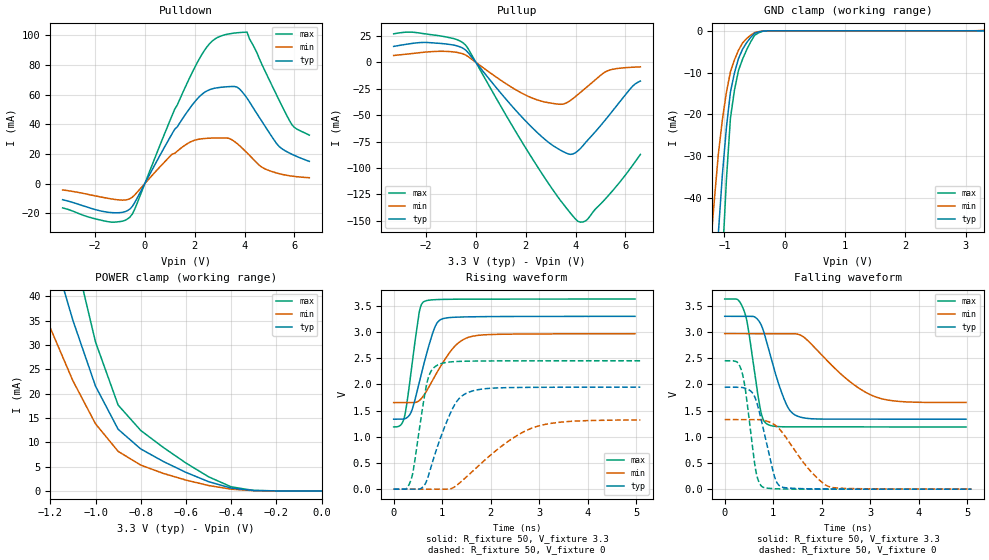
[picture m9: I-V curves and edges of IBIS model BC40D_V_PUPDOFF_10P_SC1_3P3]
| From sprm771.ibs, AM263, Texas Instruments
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|   Model Cell BC40D_V_PUPDOFF_10P_SC1_3P3
|BC40D_V_PUPDOFF_10P_SC1_3P3
[Model]   BC40D_V_PUPDOFF_10P_SC1_3P3
Model_type   I/O
Polarity   Non-Inverting
Enable   Active-Low
Vinl =  0.8V
Vinh =  2V
Cref =  15pF
Rref =  100.0000M
Vref =  0V
Vmeas =  1.65
C_comp   2.059994p   1.912853p   2.135747p
|[Input load] weak_pupdoff
|[Output drive] slow
|[supplytol] 10
|[temp] ind
[Model Spec]
Vinl   0.8V   0.8V   0.8V
Vinh   2V   2V   2V
[Temperature Range]   25   125   -40
[Voltage Range]   3.3   2.97   3.63
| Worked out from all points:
|   slope of the pulldown table from 0 to 0.495 V, typ, clamps not added: 31.8 ohm
|   slope of the pullup table from 0 to 0.495 V, typ, clamps not added: 33.8 ohm
|   GND clamp passes 1 mA (typ) near -0.53 V on its own axis
|   POWER clamp passes 1 mA (typ) near -0.43 V on its own axis
|   rising waveform, R_fixture 50, V_fixture 3.3: 20-80 % time 334ps typ, 531ps min, 209ps max; typ from 1.34 V to 3.3 V
|   rising waveform, R_fixture 50, V_fixture 0: 20-80 % time 466ps typ, 1.07ns min, 244ps max; typ from 0 V to 1.95 V
|   falling waveform, R_fixture 50, V_fixture 3.3: 20-80 % time 385ps typ, 931ps min, 234ps max; typ from 3.3 V to 1.34 V
|   falling waveform, R_fixture 50, V_fixture 0: 20-80 % time 293ps typ, 644ps min, 201ps max; typ from 1.95 V to 0 V
| Nom Voltages:
|   VDD=1.1001, VDDS=3.3, VDDS18=1.8, ESD_BIASFET=0, VSS=0, VSSS=0
| Min Voltages:
|   VDD=0.99, VDDS=2.97, VDDS18=1.62, ESD_BIASFET=0, VSS=0, VSSS=0
| Max Voltages:
|   VDD=1.21, VDDS=3.63, VDDS18=1.98, ESD_BIASFET=0, VSS=0, VSSS=0
[POWER_clamp]
|   voltage   I(typ)   I(min)   I(max)
-3.3V     446.9mA    419.5mA    603.9mA
-1.267V   62.17mA    41.5mA     88.03mA
-1.233V   56.52mA    37.5mA     80.22mA
-1.133V   40.34mA    26.27mA    57.61mA
-1.067V   30.56mA    19.7mA     43.68mA
-1.033V   26.05mA    16.75mA    37.15mA
-1V       21.55mA    13.8mA     30.62mA
-900mV    12.68mA    8.135mA    17.65mA
-800mV    8.63mA     5.309mA    12.43mA
-600mV    3.813mA    2.231mA    5.733mA
-400mV    580.7uA    357.1uA    842.6uA
0V        4.589uA    2.01uA     9.301uA
[Pulldown]
|   voltage   I(typ)   I(min)   I(max)
-3.3V     -10.93mA   -4.311mA   -16.48mA
-1.4V     -19.53mA   -10.23mA   -25.96mA
-600mV    -17.23mA   -10.26mA   -22.66mA
1.1V      33.82mA    19.89mA    46.25mA
2V        55.14mA    29.24mA    78.29mA
2.6V      63.35mA    30.61mA    94.45mA
3.2V      65.21mA    30.81mA    100.4mA
3.7V      65.09mA    27.02mA    101.8mA
4.1V      57.63mA    20.71mA    102.2mA
5.3V      26.68mA    7.058mA    59.31mA
5.9V      19.77mA    5.007mA    39.76mA
6.6V      14.97mA    3.923mA    32.7mA
[Pullup]
|   voltage   I(typ)   I(min)   I(max)
-3.3V     15.12mA    6.498mA    27.02mA
-1.9V     18.73mA    9.943mA    26.53mA
-900mV    16.4mA     9.888mA    22.58mA
-400mV    11.39mA    6.786mA    15.98mA
2.4V      -65.08mA   -35.06mA   -96.18mA
3.5V      -84.52mA   -39.53mA   -134mA
3.8V      -87.17mA   -36.01mA   -143mA
4.1V      -83.69mA   -30.35mA   -150.6mA
4.4V      -75.99mA   -24.42mA   -150.3mA
5.3V      -51.41mA   -7.872mA   -126.6mA
6.3V      -22.29mA   -4.606mA   -97.15mA
6.6V      -17.71mA   -4.277mA   -87.2mA
[GND_clamp]
|   voltage   I(typ)   I(min)   I(max)
-3.3V     -787.2mA   -607.8mA   -1.235A
-1.233V   -85.66mA   -52.14mA   -138.8mA
-1.167V   -66.47mA   -40.37mA   -107.7mA
-1.1V     -48.25mA   -29.37mA   -77.98mA
-1.033V   -34.27mA   -21.19mA   -54.56mA
-966.7mV  -23.06mA   -14.66mA   -35.51mA
-900mV    -14.61mA   -9.789mA   -20.83mA
-833.3mV  -10.05mA   -6.934mA   -14.15mA
-700mV    -4.416mA   -2.931mA   -6.811mA
-500mV    -621.6uA   -443.4uA   -1.094mA
-300mV    -17.13uA   -24.29uA   -23.57uA
3.3V      4.589uA    110.6uA    5.608uA
[Ramp]
| variable   typ   min   max
dV/dt_f  1.1805738/0.3856329n 0.79476876/0.93922811n  1.4675033/0.23410022n
dV/dt_r  1.1742366/0.46733719n 0.80289248/1.0812442n  1.4769635/0.2448637n
R_load = 50
[Rising Waveform]
R_fixture = 50
V_fixture = 3.3
V_fixture_min = 2.97
V_fixture_max = 3.63
|   time   V(typ)   V(min)   V(max)
0s        1.337V     1.652V     1.189V
223.4ps   1.343V     1.652V     1.383V
365.8ps   1.483V     1.652V     2.284V
518.8ps   2.001V     1.685V     3.334V
629.3ps   2.414V     1.802V     3.584V
806.8ps   2.985V     2.086V     3.616V
923.7ps   3.206V     2.279V     3.621V
1.266ns   3.283V     2.734V     3.627V
1.558ns   3.291V     2.904V     3.628V
4.974ns   3.3V       2.967V     3.63V
[Rising Waveform]
R_fixture = 50
V_fixture = 0
V_fixture_min = 0
V_fixture_max = 0
|   time   V(typ)   V(min)   V(max)
0s        0V         0V         0V
249.1ps   0V         0V         0V
353.3ps   0V         0V         165.9mV
568ps     16.56mV    0V         1.387V
691.3ps   186.6mV    0V         2.047V
902.7ps   815.9mV    0V         2.369V
1.273ns   1.636V     54.52mV    2.437V
1.614ns   1.872V     330.8mV    2.446V
2.938ns   1.945V     1.194V     2.451V
5.085ns   1.948V     1.321V     2.452V
[Falling Waveform]
R_fixture = 50
V_fixture = 3.3
V_fixture_min = 2.97
V_fixture_max = 3.63
|   time   V(typ)   V(min)   V(max)
0s        3.3V       2.969V     3.629V
269.7ps   3.3V       2.969V     3.617V
405.9ps   3.3V       2.969V     3.388V
482.3ps   3.3V       2.969V     3.083V
737.7ps   3.161V     2.969V     1.513V
888ps     2.729V     2.969V     1.236V
1.25ns    1.664V     2.969V     1.19V
1.51ns    1.391V     2.958V     1.189V
3.071ns   1.337V     1.776V     1.188V
4.974ns   1.336V     1.656V     1.188V
[Falling Waveform]
R_fixture = 50
V_fixture = 0
V_fixture_min = 0
V_fixture_max = 0
|   time   V(typ)   V(min)   V(max)
0s        1.947V     1.328V     2.451V
248.7ps   1.946V     1.328V     2.43V
352.3ps   1.942V     1.328V     2.245V
428.6ps   1.925V     1.328V     1.884V
640.5ps   1.713V     1.328V     355.2mV
783.9ps   1.201V     1.318V     39.26mV
1.028ns   233.9mV    1.23V      8.037mV
1.181ns   39.88mV    1.09V      4.285mV
2.165ns   3.75mV     43.76mV    0V
5.085ns   0V         2.089mV    0V
